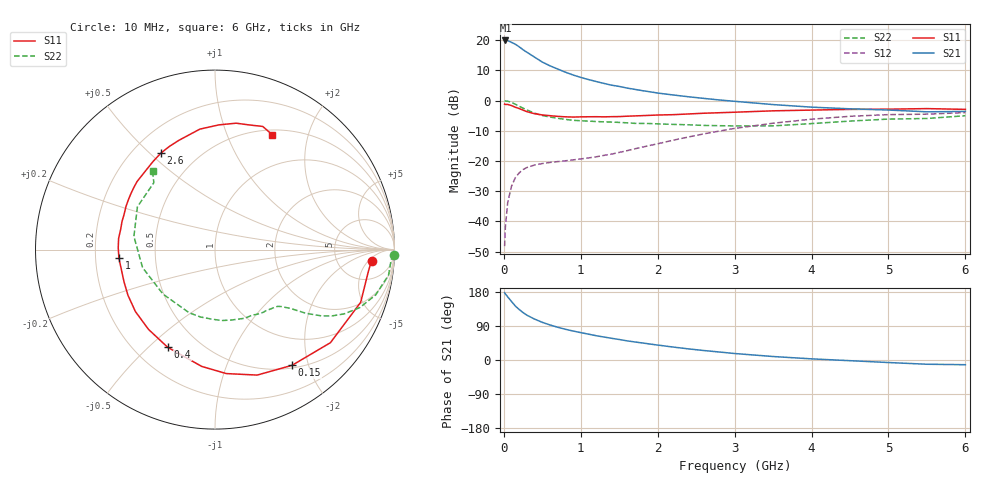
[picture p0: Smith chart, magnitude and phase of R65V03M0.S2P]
! SIEMENS Small Signal Semiconductors
! BFR193
! Si NPN RF Bipolar Junction Transistor in SOT23
! VCE = 5 V  IC = 3 mA
! Common Emitter S-Parameters:  May  1996
# GHz  S  MA  R  50
!  f  S11  S21  S12  S22
! GHz  MAG  ANG  MAG  ANG  MAG  ANG  MAG  ANG
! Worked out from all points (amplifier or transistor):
!   36 points, 10 MHz to 6 GHz, reference 50 ohm
!   highest |S21| = 19.9 dB at 20 MHz (marker M1)
!   |S21| within 3 dB of that: start of sweep to 246.1 MHz
!   unconditionally stable (mu >= 1): 1.071 GHz to 2.023 GHz
!   at 250 MHz: K = 0.30, MSG = 19.8 dB, |S12| = -22.8 dB
!   at 1.4 GHz: K = 1.10, MAG = 9.5 dB, |S12| = -17.7 dB
!   at 6 GHz: K = 0.98, MSG = 0.2 dB, |S12| = -4.0 dB
!   S11 on the Smith chart (normalised r, x): 10 MHz: 12, -6; 150 MHz: 0.54, -1.74; 400 MHz: 0.34, -0.58; 1 GHz: 0.30, -0.04; 2.6 GHz: 0.31, +0.54; 6 GHz: 0.56, +1.47
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0.01  0.8741 -4.0  9.756 177.6  0.0039 91.0  0.9956 -1.6
0.02  0.8633 -8.0  9.869 174.5  0.0081 87.7  0.983 -3.3
0.05  0.8631 -19.9  9.82 166.6  0.0205 79.4  0.9775 -8.3
0.1  0.8261 -38.9  9.174 154.4  0.0384 70.3  0.9306 -15.7
0.15  0.7747 -56.3  8.544 142.3  0.0531 62.0  0.8693 -21.8
0.2  0.7376 -71.4  7.742 133.1  0.0637 55.6  0.8047 -26.4
0.25  0.6936 -84.8  6.926 125.1  0.0722 50.5  0.7485 -29.6
0.3  0.655 -96.5  6.297 118.2  0.0781 47.1  0.6991 -31.9
0.4  0.6048 -115.8  5.22 107.9  0.0858 42.5  0.6189 -35.0
0.5  0.5787 -129.8  4.331 99.4  0.0908 40.3  0.5663 -36.7
0.6  0.5619 -142.1  3.756 92.5  0.0946 39.6  0.5338 -37.9
0.7  0.5477 -152.3  3.324 86.4  0.0978 40.1  0.5089 -39.3
0.8  0.5379 -160.4  2.948 81.1  0.1008 41.4  0.4879 -40.6
1  0.5376 -174.8  2.412 72.2  0.1083 45.3  0.4632 -43.8
1.1  0.5392 178.8  2.226 68.2  0.1124 47.5  0.4566 -45.8
1.6  0.551 154.2  1.611 50.6  0.148 57.2  0.4283 -57.6
2.2  0.5842 131.9  1.238 34.2  0.2208 60.8  0.4033 -76.5
2.6  0.617 119.1  1.086 25.0  0.2811 58.2  0.3877 -92.8
3.5  0.6764 97.2  0.858 9.2  0.4219 44.6  0.3814 -139.4
4.5  0.7141 80.5  0.73 -1.8  0.5491 25.8  0.4577 170.8
5.5  0.7359 68.8  0.651 -11.2  0.5958 7.1  0.5052 132.4
6  0.7148 63.4  0.661 -12.4  0.6326 1.9  0.5613 128.3
